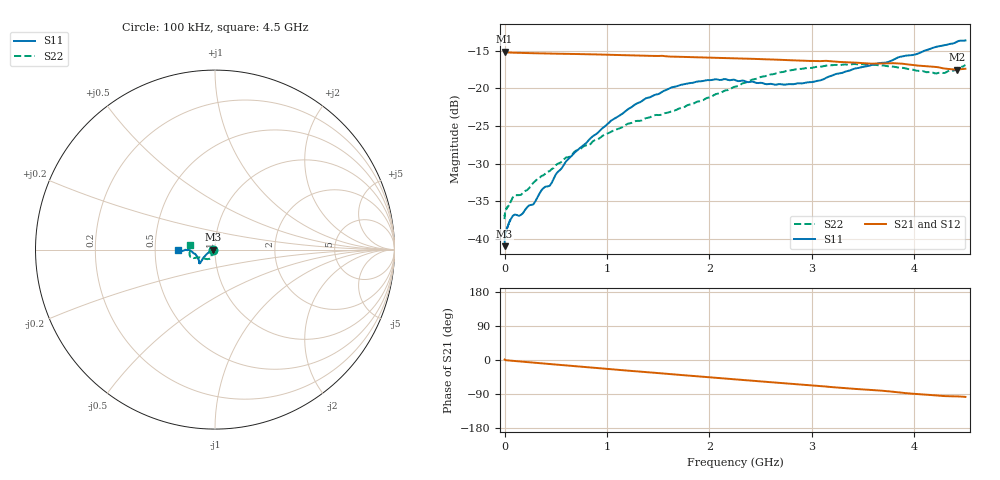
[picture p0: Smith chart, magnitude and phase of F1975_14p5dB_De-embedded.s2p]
! Integrated Device Technology
! Corporate Headquarters
! 6024 Silver Creek Valley Road
! San Jose, CA 95138  USA
! Phone:  1-408-284-8200
! Toll Free:  1-800-223-1366
! Webpage:  http://www.idt.com/
! Timing and RF Division
! 515 Groton Road, Suite 102
! Westford, MA 01886-6024
! Device:  F1975
! Description: 6-bit, 75 ohm, 0.5 dB Digital Step Attenuator
! Frequency:  5.0 MHz -  3.00 GHz
! Package:  4x4 mm QFN Plastic Package: 20 pin
! Ports:  2 RF, 11 DC
!  Pin  1  = D5 (16 dB)
!  Pin  2  = RF1  =  Port 1
!  Pin  3  = Serial Data In (DATA)
!  Pin  4  = Serial Clock (CLK)
!  Pin  5  = Serial Latch Enable (LE)
!  Pin  6  = VDD
!  Pin  7  = NC
!  Pin  8  = NC
!  Pin  9  = NC
!  Pin 10  = GND
!  Pin 11  = GND
!  Pin 12  = NC
!  Pin 13  = VMODE
!  Pin 14  = RF2  =  Port 2
!  Pin 15  = D4 (8 dB)
!  Pin 16  = D3 (4 dB)
!  Pin 17  = D2 (2 dB)
!  Pin 18  = NC
!  Pin 19  = D1 (1 dB)
!  Pin 20  = D0 (0.5 dB)
! State:  29
! Atten State:  14.5 dB
! Voltage:  +3.30 Volts
! Current:  0.565 mA
! Data:  The device was measured on a F1975 evaluation board which has
!  individual transmission lines to the RF pins.  Data was collected
!  using a calibrated network analyzer.  The evaluation board was
!  de-embedded using Automatic Fixture Removal (AFR).
!  The reference plane is the edge of the package pin.
! Misc:
!  Action Tracker AT0415
! Date Measured:  2018-02-08
! Date:  2018-03-26  MJV
! Note:
!  Integrated Device Technology supplies this data as a sample of measured
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# GHz S dB R 75
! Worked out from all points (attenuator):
!   291 points, 100 kHz to 4.5 GHz, reference 75 ohm
!   highest |S21| = -15.11 dB at 100 kHz (marker M1); lowest = -17.5 dB at 4.42 GHz (marker M2)
!   lowest |S11| = -41.0 dB at 100 kHz (marker M3), VSWR 1.02, Z = 73.7 - j0.00382 ohm
!   |S11| at or under -10 dB: start of sweep to end of sweep
!   |S22| runs from -37.4 to -16.7 dB; largest |S21 - S12| = 0.00013
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0.0001  -41.00 -179.8  -15.11 1.2  -15.11 1.2  -37.39 -178.7
0.0006  -40.07 -176.9  -15.13 1.1  -15.13 1.1  -36.98 -177.6
0.003  -39.57 -176.8  -15.15 0.7  -15.16 0.7  -36.55 -176.9
0.014  -38.90 -174.4  -15.19 -0.6  -15.19 -0.6  -36.10 -173.4
0.08  -36.96 -168.5  -15.23 -2.2  -15.23 -2.2  -34.50 -162.3
0.16  -36.83 -165.1  -15.27 -4.1  -15.27 -4.1  -34.16 -147.2
0.28  -35.44 -164.3  -15.30 -6.9  -15.30 -6.9  -32.55 -136.7
0.36  -33.57 -164.2  -15.33 -8.8  -15.32 -8.8  -31.65 -128.8
0.44  -32.97 -161.9  -15.34 -10.6  -15.34 -10.6  -31.01 -123.2
0.6  -29.71 -160.1  -15.39 -14.3  -15.39 -14.3  -29.19 -119.8
0.76  -27.67 -154.4  -15.43 -17.9  -15.43 -17.9  -27.83 -118.0
1.04  -24.28 -149.3  -15.51 -24.4  -15.51 -24.4  -25.76 -117.7
1.38  -21.31 -143.6  -15.64 -32.0  -15.64 -32.0  -23.94 -124.2
1.52  -20.62 -140.6  -15.66 -35.0  -15.65 -35.0  -23.53 -128.0
1.88  -19.08 -138.0  -15.85 -42.9  -15.84 -42.9  -21.76 -143.1
2.26  -18.93 -140.2  -15.98 -51.2  -15.97 -51.2  -19.73 -154.5
2.64  -19.50 -150.8  -16.15 -59.4  -16.15 -59.4  -18.04 -158.2
3.02  -19.10 -165.9  -16.34 -67.3  -16.33 -67.3  -17.19 -161.6
3.76  -16.40 -178.9  -16.63 -82.8  -16.62 -82.8  -17.05 -175.0
4.2  -14.51 -177.7  -17.12 -93.3  -17.12 -93.3  -17.98 173.4
4.42  -13.75 -177.1  -17.47 -96.1  -17.47 -96.1  -17.31 170.2
4.5  -13.60 -179.0  -17.37 -97.4  -17.37 -97.4  -16.86 169.1
